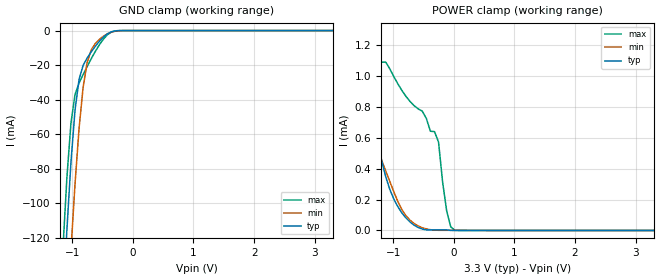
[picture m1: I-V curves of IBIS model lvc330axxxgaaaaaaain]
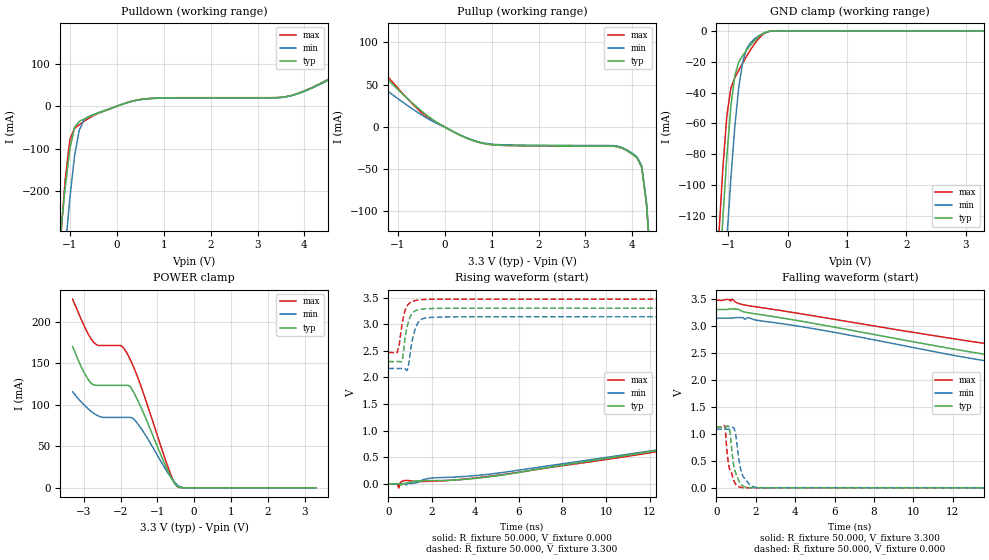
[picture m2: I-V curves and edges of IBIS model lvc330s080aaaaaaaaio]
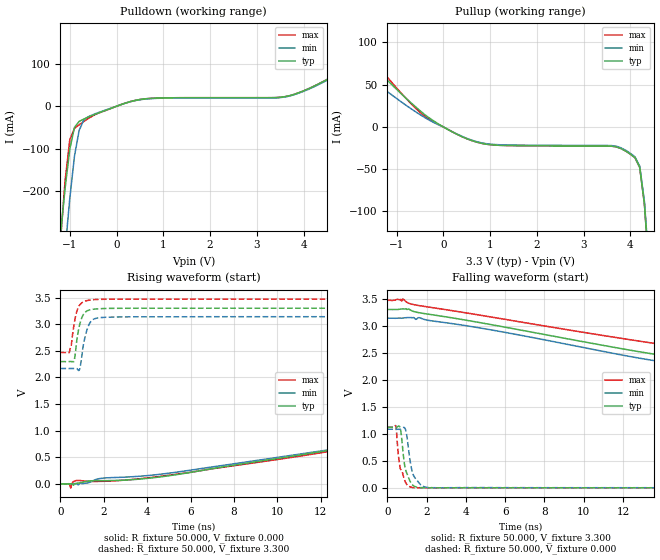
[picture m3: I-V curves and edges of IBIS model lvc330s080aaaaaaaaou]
| IBIS Models Generator: Lattice Radiant Software (64-bit) 3.2.1.217.3
| Report Generate Date: Nov 11 2022
| Report Generate Time: 17:06:55
| IBIS File LibisMaker.ibs
| Cadence Design Systems, Inc. 2021
[IBIS ver]   4.2
[File Name]   Lab1_impl_1.ibs
[File Rev]   1.0
[Date]   Wed Dec  1 00:22:15 PST 2021
[Source]   Lattice Semiconductor 28fdsoi Process
[Notes]   Device: LFMXO5-25   Preliminary
   Lattice Semiconductor has worked hard to ensure the
   models below are accurate and complete.  However, the
   data below was generated using simulation of the
   input/output model files for the silicon.  Therefore,
   the data below is for reference and initial design
   purposes only.
   Lattice Semiconductor grants permission to use this
   data for use in printed circuit design using this
   Lattice programmable logic device.  Other use of this
   code, including the selling or duplication of any
   portion is strictly prohibited.
|   NAMING CONVENTION
   The IBIS [Model] header is limited by the specification to a
   total of characters.  With such a set of characters available
   for naming models it becomes important to attempt to
   meaningfully encode the IO standards so they fit within the
   twenty character limit.  It would seem that twenty characters
   would provide room enough for describing IO's.  However, the
   PLD IO structure continues to grow more and more complex.  The
   complexity is making the twenty characters insuffiently
   descriptive.  In order to overcome this issue the naming
   convention described below is implemented to resolve the issue.
The twenty character space is managed as follows:
   bbbvvvsdddprttmaoixx
   b = standard
   v = voltage (x.xx V)
   s = slew code
   d = drive (xx.x ma)
   p = pullmode code
   r = impedance
   t = termination code
   m = mipi hard dphy mode
   o = diff resistor code
   i = diff  current code
   x = reserved
   standard
   LVCMOS   lvc
   LVCMOSH   lvh
   LVCMOSR   lvr
   I3C   i3c
   LVCMOSD   lvd
   LVTTL   lvt
   lvttld   ltd
   sstl_I   ss1
   sstl_II   ss2
   sstld_I   s1d
   sstld_II   s2d
   hsul   hs1
   hsuld   h1d
   hstl_I   hs1
   hstld_I   h1d
   lvds   lvs
   lvdse   lve
   SUBLVDS   slv
   sublvdse   sle
   sublvdseh   slh
   slvs   svs
   mipi   mip
   vref1   vr1
   slew
   na   a
   fast   f
   slow   s
   med   m
   drive
   2   020
   4   040
   6   060
   8   080
   10   100
   12   120
   16   160
   50rs   r50
   na   xxx
   pullmode/clamp on
   none   a/e
   failsafe   a/e
   up   b/f
   down   c/g
   keeper   d/h
   i3c   i
   impedance
   off   a
   termination
   off   aa
   40   bb
   50   cc
   60   dd
   75   ee
   150   ff
   mipi hard dphy mode
   off   a
   lp   l
   hs   h
   differential resistor
   off   a
   100   b
   differential current
   NA   a
   2.0   b
   3.5   c
   Reserved   IO type
   in   input only (mipi: rx)
   ou   output (mipi: tx)
   io   I/O
   od   Open drain
   on   Inverting differential I/O
   op   Non-Inverting differential I/O
   All the IO models are generated with pull mode set to none.
   Lattice Semiconductor Corporation
   5555 NE Moore Court
   Hillsboro, OR 97214
   U.S.A
   TEL: 1-800-Lattice (USA and Canada)
   408-826-6000 (other locations)
   web: http://www.latticesemi.com/
   email: techsupport@latticesemi.com
[Disclaimer] This IBIS source code is intended as a design reference
   which illustrates how the Lattice Semiconductor device operates.
   It is the user's responsibility to verify their design for
   consistency and functionality through the use of formal
   verification methods.  Lattice Semiconductor provides no warranty
   regarding the use or functionality of this data.
[Copyright]   Copyright 2021 by Lattice Semiconductor Corporation
|   Component LFMXO5
[Component] LFMXO5
[Manufacturer] Lattice Semiconductor Corp.
[Package]
|BBG400
| variable   typ   min   max
R_pkg   0.36549   0.21269   0.57866
L_pkg   3.644e-9   2.134e-9   6.024e-9
C_pkg   1.195e-12   7.084e-13   1.745e-12
[Pin]  signal_name   model_name   R_pin   L_pin   C_pin
E18   TDI   lvc330axxxgaaaaaaain
G16   TCK   lvc330axxxgaaaaaaain
F16   TMS   lvc330axxxgaaaaaaain
E20   TDO   lvc330s080aaaaaaaaio
A18   SEG_OUT[7]   lvc330s080aaaaaaaaou
A17   SEG_OUT[6]   lvc330s080aaaaaaaaou
A16   SEG_OUT[5]   lvc330s080aaaaaaaaou
A15   SEG_OUT[4]   lvc330s080aaaaaaaaou
F11   SEG_OUT[3]   lvc330s080aaaaaaaaou
E15   SEG_OUT[2]   lvc330s080aaaaaaaaou
G11   SEG_OUT[1]   lvc330s080aaaaaaaaou
F14   SEG_OUT[0]   lvc330s080aaaaaaaaou
G12   LED_OUT[7]   lvc330s080aaaaaaaaou
G13   LED_OUT[6]   lvc330s080aaaaaaaaou
H11   LED_OUT[5]   lvc330s080aaaaaaaaou
H12   LED_OUT[4]   lvc330s080aaaaaaaaou
P7   LED_OUT[3]   lvc330s080aaaaaaaaou
R1   LED_OUT[2]   lvc330s080aaaaaaaaou
R2   LED_OUT[1]   lvc330s080aaaaaaaaou
R3   LED_OUT[0]   lvc330s080aaaaaaaaou
A4   MON[3]   lvc330s080aaaaaaaaou
C2   MON[2]   lvc330s080aaaaaaaaou
C3   MON[1]   lvc330s080aaaaaaaaou
E4   MON[0]   lvc330s080aaaaaaaaou
D3   ROM_OUT[17]   lvc330s080aaaaaaaaou
H13   ROM_OUT[16]   lvc330s080aaaaaaaaou
J12   ROM_OUT[15]   lvc330s080aaaaaaaaou
J14   ROM_OUT[14]   lvc330s080aaaaaaaaou
J13   ROM_OUT[13]   lvc330s080aaaaaaaaou
J16   ROM_OUT[12]   lvc330s080aaaaaaaaou
J15   ROM_OUT[11]   lvc330s080aaaaaaaaou
J18   ROM_OUT[10]   lvc330s080aaaaaaaaou
J17   ROM_OUT[9]   lvc330s080aaaaaaaaou
H19   ROM_OUT[8]   lvc330s080aaaaaaaaou
H20   ROM_OUT[7]   lvc330s080aaaaaaaaou
G19   ROM_OUT[6]   lvc330s080aaaaaaaaou
H16   ROM_OUT[5]   lvc330s080aaaaaaaaou
G18   ROM_OUT[4]   lvc330s080aaaaaaaaou
H15   ROM_OUT[3]   lvc330s080aaaaaaaaou
G14   ROM_OUT[2]   lvc330s080aaaaaaaaou
H14   ROM_OUT[1]   lvc330s080aaaaaaaaou
C20   ROM_OUT[0]   lvc330s080aaaaaaaaou
T3   SW[2]   lvc330axxxgaaaaaaain
T2   SW[1]   lvc330axxxgaaaaaaain
T1   SW[0]   lvc330axxxgaaaaaaain
| Models and submodels in the file (3): lvc330axxxgaaaaaaain (Input), lvc330s080aaaaaaaaio (I/O), lvc330s080aaaaaaaaou (Output)
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[Model] lvc330axxxgaaaaaaain
Model_type Input
Polarity   Non-Inverting
Enable   Active-High
Vinl =  0.800V
Vinh =  2.000V
C_comp   5.000pF   4.000pF   5.500pF
[Temperature Range]   25.000   0.125k   -40.000
[Voltage Range]   3.300V   3.140V   3.470V
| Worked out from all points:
|   GND clamp passes 1 mA (typ) near -0.37 V on its own axis
|   POWER clamp passes 1 mA (typ) near -1.47 V on its own axis
[GND_clamp]
|Voltage   I(typ)   I(min)   I(max)
-3.3V     -1.865A    -1.847A    -1.883A
-1.156V   -160.1mA   -214.1mA   -127.6mA
-1.089V   -115.7mA   -169.6mA   -85.35mA
-1.022V   -76.45mA   -127.5mA   -53.7mA
-955mV    -46.24mA   -89.13mA   -37.05mA
-888mV    -28.3mA    -56.66mA   -30.41mA
-821mV    -20.19mA   -32.82mA   -25.49mA
-754mV    -15.89mA   -18.49mA   -20.81mA
-620mV    -9.094mA   -7.515mA   -12.09mA
-419mV    -1.868mA   -1.846mA   -2.383mA
-218mV    -16.48uA   -78.61uA   -6.639uA
3.3V      0A         0A         0A
[POWER_clamp]
|Voltage   I(typ)   I(min)   I(max)
-3.3V     37.53mA    9.364mA    73.7mA
-1.792V   1.823mA    1.318mA    2.466mA
-1.591V   1.29mA     991.8uA    1.714mA
-1.457V   981.8uA    795.4uA    1.299mA
-1.39V    843.7uA    703.6uA    1.091mA
-1.122V   347.7uA    385.2uA    1.091mA
-854mV    112.9uA    134.5uA    907uA
-586mV    19.15uA    28.85uA    788.2uA
-251mV    3.861uA    1.254uA    573.3uA
-117mV    3.861uA    1.254uA    126.7uA
17mV      69.96nA    1.254uA    1.636uA
3.3V      0A         0A         0A
[Model] lvc330s080aaaaaaaaio
Model_type I/O
Polarity   Non-Inverting
Enable   Active-Low
Vinl =  0.800V
Vinh =  2.000V
Vmeas =  1.650V
Cref =  0.0F
Rref =  1.000M
Vref =  0.0V
C_comp   5.000pF   4.000pF   5.500pF
[Temperature Range]   25.000   0.125k   -40.000
[Voltage Range]   3.300V   3.140V   3.470V
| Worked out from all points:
|   slope of the pulldown table from 0 to 0.495 V, typ, clamps not added: 31.5 ohm
|   slope of the pullup table from 0 to 0.495 V, typ, clamps not added: 35.9 ohm
|   GND clamp passes 1 mA (typ) near -0.37 V on its own axis
|   POWER clamp passes 1 mA (typ) near -0.42 V on its own axis
|   rising waveform, R_fixture 50.000, V_fixture 0.000: 20-80 % time 10.1ns typ, 10.8ns min, 10.1ns max; typ from 0 V to 1.12 V
|   rising waveform, R_fixture 50.000, V_fixture 3.300: 20-80 % time 265ps typ, 295ps min, 259ps max; typ from 2.3 V to 3.3 V
|   falling waveform, R_fixture 50.000, V_fixture 3.300: 20-80 % time 9.12ns typ, 8.53ns min, 10.2ns max; typ from 3.3 V to 2.3 V
|   falling waveform, R_fixture 50.000, V_fixture 0.000: 20-80 % time 306ps typ, 322ps min, 315ps max; typ from 1.12 V to 0 V
[GND_clamp]
|Voltage   I(typ)   I(min)   I(max)
-3.3V     -1.887A    -1.873A    -1.902A
-1.156V   -166.9mA   -224mA     -132.1mA
-1.089V   -121.5mA   -178.4mA   -88.64mA
-1.022V   -81.05mA   -135.2mA   -54.94mA
-955mV    -48.98mA   -95.79mA   -37.15mA
-888mV    -28.98mA   -62.05mA   -30.42mA
-821mV    -20.23mA   -36.35mA   -25.49mA
-754mV    -15.89mA   -19.89mA   -20.81mA
-687mV    -12.34mA   -11.44mA   -16.31mA
-620mV    -9.094mA   -7.515mA   -12.09mA
-419mV    -1.869mA   -1.836mA   -2.383mA
3.3V      0A         0A         0A
[POWER_clamp]
|Voltage   I(typ)   I(min)   I(max)
-3.3V     170.3mA    115.9mA    227.4mA
-2.998V   139.6mA    100.3mA    196.3mA
-2.797V   125.9mA    92.2mA     179.4mA
-2.596V   123.5mA    86.45mA    171.5mA
-1.993V   123.5mA    84.93mA    171.5mA
-1.792V   123.5mA    84.93mA    159.6mA
-1.658V   116.4mA    83.68mA    147.1mA
-1.457V   98.28mA    72.65mA    124.1mA
-720mV    21.08mA    18.41mA    25.96mA
-452mV    1.573mA    3.148mA    1.229mA
-184mV    5.589uA    37.85uA    1.612uA
3.3V      0A         0A         0A
[Pulldown]
|Voltage   I(typ)   I(min)   I(max)
-3.3V     -3.025A    -3.614A    -3.918A
-1.2V     -304.3mA   -472.8mA   -317.2mA
-1.1V     -192.9mA   -339.3mA   -175.3mA
-1V       -101.2mA   -217mA     -78.95mA
-900mV    -49.86mA   -117.7mA   -52.21mA
-800mV    -35.81mA   -56.74mA   -43.74mA
-500mV    -20.71mA   -19.76mA   -22.12mA
600mV     17.27mA    16.75mA    17.27mA
3.7V      24.69mA    23.95mA    24.69mA
5.3V      109.4mA    106.1mA    109.4mA
6.1V      131.6mA    127.7mA    131.6mA
6.6V      184.5mA    179mA      184.5mA
[Pullup]
|Voltage   I(typ)   I(min)   I(max)
-3.3V     145.5mA    90.7mA     185.8mA
-3V       114.9mA    81.5mA     156.2mA
-2.7V     96.8mA     74.7mA     125.4mA
-2.4V     95.1mA     71.05mA    105.4mA
-1.9V     90.5mA     66.84mA    102.4mA
-500mV    19.13mA    14.57mA    17.21mA
600mV     -16.01mA   -15.53mA   -16.01mA
3.8V      -25.54mA   -24.77mA   -25.54mA
4.2V      -47.87mA   -46.43mA   -47.87mA
4.3V      -90.8mA    -88.1mA    -90.8mA
4.4V      -169.3mA   -164.2mA   -169.3mA
6.6V      -2.624A    -2.545A    -2.624A
[Ramp]
| variable   typ   min   max
dV/dt_r   0.690/10.154n   0.471/10.738n   0.489/10.105n
dV/dt_f   0.678/9.145n   0.512/8.567n   0.500/10.251n
R_load = 50.000
[Rising Waveform]
R_fixture = 50.000
V_fixture = 0.000
V_fixture_min = 0.000
V_fixture_max = 0.000
|  time   V(typ)   V(min)   V(max)
0s        488.9uV    1.45mV     490.1uV
395ps     658.9uV    837.7uV    4.122mV
476ps     748.1uV    1.464mV    -75.06mV
567ps     -9.748mV   1.636mV    30.57mV
756ps     9.529mV    3.994mV    63.46mV
1.276ns   53.06mV    19.22mV    47.44mV
1.915ns   60.52mV    105.6mV    47.56mV
4.871ns   145.2mV    193.8mV    154.5mV
18.34ns   1.028V     996.8mV    1.045V
20ns      1.119V     1.084V     1.122V
[Rising Waveform]
R_fixture = 50.000
V_fixture = 3.300
V_fixture_min = 3.140
V_fixture_max = 3.470
|  time   V(typ)   V(min)   V(max)
0s        2.297V     2.167V     2.467V
409ps     2.297V     2.166V     2.466V
495ps     2.298V     2.167V     2.59V
617ps     2.297V     2.168V     2.964V
732ps     2.615V     2.168V     3.208V
866ps     2.954V     2.137V     3.345V
1.122ns   3.215V     2.737V     3.43V
1.393ns   3.272V     3.045V     3.454V
2.705ns   3.298V     3.135V     3.469V
20ns      3.3V       3.14V      3.47V
[Falling Waveform]
R_fixture = 50.000
V_fixture = 3.300
V_fixture_min = 3.140
V_fixture_max = 3.470
|  time   V(typ)   V(min)   V(max)
0s        3.3V       3.14V      3.47V
688ps     3.308V     3.14V      3.488V
728ps     3.309V     3.14V      3.458V
798ps     3.311V     3.142V     3.492V
1.104ns   3.305V     3.151V     3.415V
1.456ns   3.252V     3.118V     3.382V
1.635ns   3.24V      3.148V     3.371V
14.38ns   2.432V     2.313V     2.632V
17.15ns   2.336V     2.218V     2.518V
20ns      2.297V     2.167V     2.467V
[Falling Waveform]
R_fixture = 50.000
V_fixture = 0.000
V_fixture_min = 0.000
V_fixture_max = 0.000
|  time   V(typ)   V(min)   V(max)
0s        1.119V     1.084V     1.122V
432ps     1.119V     1.083V     1.146V
635ps     1.128V     1.083V     409.9mV
704ps     1.006V     1.09V      325.8mV
894ps     392.5mV    1.102V     128.6mV
976ps     284.1mV    1.002V     70.9mV
1.286ns   53.13mV    272.9mV    6.472mV
1.736ns   2.839mV    45mV       -634.6uV
2.289ns   60.46uV    2.35mV     -755.8uV
20ns      488.9uV    1.45mV     490.1uV
[Model] lvc330s080aaaaaaaaou
Model_type Output
Polarity   Non-Inverting
Enable   Active-High
Vmeas =  1.650V
Cref =  0.0F
Rref =  1.000M
Vref =  0.0V
C_comp   5.000pF   4.000pF   5.500pF
[Temperature Range]   25.000   0.125k   -40.000
[Voltage Range]   3.300V   3.140V   3.470V
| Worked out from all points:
|   slope of the pulldown table from 0 to 0.495 V, typ, clamps not added: 31.5 ohm
|   slope of the pullup table from 0 to 0.495 V, typ, clamps not added: 35.9 ohm
|   rising waveform, R_fixture 50.000, V_fixture 0.000: 20-80 % time 10.1ns typ, 10.8ns min, 10.1ns max; typ from 0 V to 1.12 V
|   rising waveform, R_fixture 50.000, V_fixture 3.300: 20-80 % time 265ps typ, 295ps min, 259ps max; typ from 2.3 V to 3.3 V
|   falling waveform, R_fixture 50.000, V_fixture 3.300: 20-80 % time 9.12ns typ, 8.53ns min, 10.2ns max; typ from 3.3 V to 2.3 V
|   falling waveform, R_fixture 50.000, V_fixture 0.000: 20-80 % time 306ps typ, 322ps min, 315ps max; typ from 1.12 V to 0 V
[Pulldown]
|Voltage   I(typ)   I(min)   I(max)
-3.3V     -3.025A    -3.614A    -3.918A
-1.2V     -304.3mA   -472.8mA   -317.2mA
-1.1V     -192.9mA   -339.3mA   -175.3mA
-1V       -101.2mA   -217mA     -78.95mA
-900mV    -49.86mA   -117.7mA   -52.21mA
-800mV    -35.81mA   -56.74mA   -43.74mA
-500mV    -20.71mA   -19.76mA   -22.12mA
600mV     17.27mA    16.75mA    17.27mA
3.7V      24.69mA    23.95mA    24.69mA
5.3V      109.4mA    106.1mA    109.4mA
6.1V      131.6mA    127.7mA    131.6mA
6.6V      184.5mA    179mA      184.5mA
[Pullup]
|Voltage   I(typ)   I(min)   I(max)
-3.3V     145.5mA    90.7mA     185.8mA
-3V       114.9mA    81.5mA     156.2mA
-2.7V     96.8mA     74.7mA     125.4mA
-2.4V     95.1mA     71.05mA    105.4mA
-1.9V     90.5mA     66.84mA    102.4mA
-500mV    19.13mA    14.57mA    17.21mA
600mV     -16.01mA   -15.53mA   -16.01mA
3.8V      -25.54mA   -24.77mA   -25.54mA
4.2V      -47.87mA   -46.43mA   -47.87mA
4.3V      -90.8mA    -88.1mA    -90.8mA
4.4V      -169.3mA   -164.2mA   -169.3mA
6.6V      -2.624A    -2.545A    -2.624A
[Ramp]
| variable   typ   min   max
dV/dt_r   0.690/10.154n   0.471/10.738n   0.489/10.105n
dV/dt_f   0.678/9.145n   0.512/8.567n   0.500/10.251n
R_load = 50.000
[Rising Waveform]
R_fixture = 50.000
V_fixture = 0.000
V_fixture_min = 0.000
V_fixture_max = 0.000
|  time   V(typ)   V(min)   V(max)
0s        488.9uV    1.443mV    488.9uV
395ps     658.9uV    831.3uV    4.121mV
476ps     748.1uV    1.458mV    -75.06mV
567ps     -9.748mV   1.629mV    30.57mV
756ps     9.529mV    3.988mV    63.46mV
1.276ns   53.06mV    19.21mV    47.44mV
1.915ns   60.52mV    105.6mV    47.56mV
4.871ns   145.2mV    193.8mV    154.5mV
18.34ns   1.028V     996.8mV    1.045V
20ns      1.119V     1.084V     1.122V
[Rising Waveform]
R_fixture = 50.000
V_fixture = 3.300
V_fixture_min = 3.140
V_fixture_max = 3.470
|  time   V(typ)   V(min)   V(max)
0s        2.297V     2.167V     2.467V
409ps     2.297V     2.166V     2.466V
495ps     2.298V     2.167V     2.59V
617ps     2.297V     2.168V     2.964V
732ps     2.615V     2.168V     3.208V
866ps     2.954V     2.137V     3.345V
1.122ns   3.215V     2.737V     3.43V
1.393ns   3.272V     3.045V     3.454V
2.705ns   3.298V     3.135V     3.469V
20ns      3.3V       3.14V      3.47V
[Falling Waveform]
R_fixture = 50.000
V_fixture = 3.300
V_fixture_min = 3.140
V_fixture_max = 3.470
|  time   V(typ)   V(min)   V(max)
0s        3.3V       3.14V      3.47V
688ps     3.308V     3.14V      3.488V
728ps     3.309V     3.14V      3.458V
798ps     3.311V     3.142V     3.492V
1.104ns   3.305V     3.151V     3.415V
1.456ns   3.252V     3.118V     3.382V
1.635ns   3.24V      3.148V     3.371V
14.38ns   2.432V     2.313V     2.632V
17.15ns   2.336V     2.218V     2.518V
20ns      2.297V     2.167V     2.467V
[Falling Waveform]
R_fixture = 50.000
V_fixture = 0.000
V_fixture_min = 0.000
V_fixture_max = 0.000
|  time   V(typ)   V(min)   V(max)
0s        1.119V     1.084V     1.122V
432ps     1.119V     1.083V     1.146V
635ps     1.128V     1.083V     409.9mV
704ps     1.006V     1.09V      325.8mV
894ps     392.5mV    1.102V     128.6mV
976ps     284.1mV    1.002V     70.9mV
1.286ns   53.13mV    272.9mV    6.471mV
1.736ns   2.839mV    45mV       -635.9uV
2.289ns   60.46uV    2.344mV    -757.1uV
20ns      488.9uV    1.443mV    488.9uV
